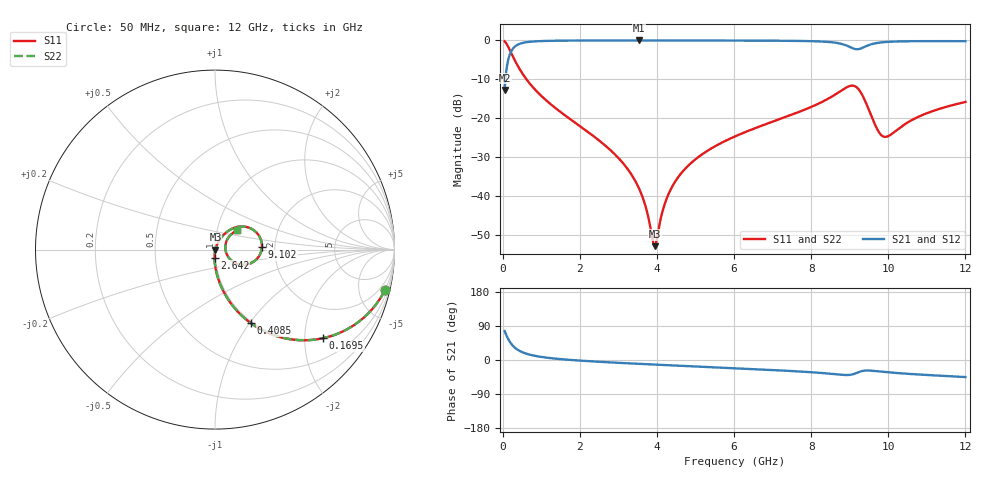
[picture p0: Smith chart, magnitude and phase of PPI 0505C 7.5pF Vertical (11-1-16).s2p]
# GHz S MA R 50
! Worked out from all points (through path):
!   1601 points, 50 MHz to 12 GHz, reference 50 ohm
!   highest |S21| = -0.02 dB at 3.53 GHz (marker M1); lowest = -12.7 dB at 50 MHz (marker M2)
!   group delay of S21, straight-line fit = 14.3 ps
!   lowest |S11| = -52.8 dB at 3.941 GHz (marker M3), VSWR 1.00, Z = 50.2 - j0.0466 ohm
!   |S11| at or under -10 dB: 618 MHz to end of sweep
!   |S22| runs from -52.8 to -0.2 dB; largest |S21 - S12| = 0
!   S11 on the Smith chart (normalised r, x): 50 MHz: 0.98, -8.34; 169.5 MHz: 0.98, -2.46; 408.5 MHz: 0.98, -1.01; 2.642 GHz: 0.99, -0.09; 9.102 GHz: 1.71, +0.05; 12 GHz: 1.24, +0.27
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0.05  0.973 -13.5  0.2306 76.5  0.2306 76.5  0.973 -13.5
0.1695  0.7788 -39.3  0.6268 50.6  0.6268 50.6  0.7788 -39.3
0.4085  0.455 -64.1  0.8897 25.8  0.8897 25.8  0.455 -64.1
0.8715625  0.225 -79.4  0.9732 10.3  0.9732 10.3  0.225 -79.4
2.044156  0.0769 -90.7  0.9953 -1.9  0.9953 -1.9  0.0769 -90.7
2.641656  0.04566 -93.2  0.9969 -5.5  0.9969 -5.5  0.04566 -93.2
3.171937  0.02483 -93.6  0.9975 -8.3  0.9975 -8.3  0.02483 -93.6
3.530438  0.01282 -90.4  0.9975 -10.1  0.9975 -10.1  0.01282 -90.4
3.702219  0.007553 -83.9  0.9975 -10.9  0.9975 -10.9  0.007553 -83.9
3.941219  0.0023 -11.6  0.9974 -12.1  0.9974 -12.1  0.0023 -11.6
4.038312  0.003705 38.4  0.9974 -12.5  0.9974 -12.5  0.003705 38.4
4.269844  0.009847 62.1  0.9973 -13.6  0.9973 -13.6  0.009847 62.1
4.628344  0.01974 67.3  0.9969 -15.3  0.9969 -15.3  0.01974 67.3
6.025  0.05872 64.9  0.9945 -21.7  0.9945 -21.7  0.05872 64.9
8.019156  0.1414 52.3  0.9764 -32.4  0.9764 -32.4  0.1414 52.3
8.766031  0.2244 33.1  0.9067 -38.8  0.9067 -38.8  0.2244 33.1
9.102125  0.2618 3.0  0.7848 -37.1  0.7848 -37.1  0.2618 3.0
9.356063  0.1861 -27.0  0.8134 -28.4  0.8134 -28.4  0.1861 -27.0
9.766844  0.06554 -16.7  0.9355 -30.2  0.9355 -30.2  0.06554 -16.7
10.01331  0.05969 15.9  0.9588 -32.6  0.9588 -32.6  0.05969 15.9
10.84234  0.1082 42.7  0.9771 -38.6  0.9771 -38.6  0.1082 42.7
12  0.1623 41.3  0.9756 -45.0  0.9756 -45.0  0.1623 41.3
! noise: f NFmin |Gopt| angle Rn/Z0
0.05  0.000457  0.8904  1.895  0.0009076
1.372  0.004385  0.6995  4.729  0.00285
2.701  0.007223  0.6515  8.53  0.00392
4.031  0.009861  0.6262  12.33  0.004884
5.36  0.01274  0.6188  16.1  0.006115
6.682  0.01719  0.6444  19.87  0.008891
8.012  0.03233  0.7592  23.93  0.02605
9.341  0.1457  0.9321  28.11  0.4491
10.67  0.04421  0.7681  31.73  0.03596
12  0.03525  0.6904  35.03  0.02022
